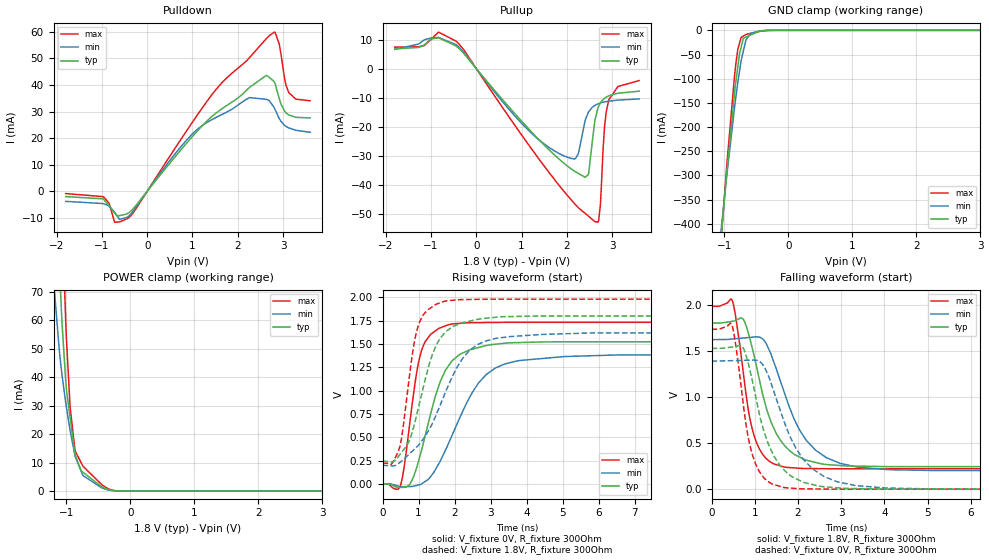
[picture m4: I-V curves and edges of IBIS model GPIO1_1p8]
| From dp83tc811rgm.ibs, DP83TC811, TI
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|   GPIO1_1p8 Model
[Model]   GPIO1_1p8
Model_type   I/O
Polarity   Non-Inverting
Enable   Active-Low
Vinl = 0.63
Vinh = 1.17
Vmeas = 0.9
Vref = 0
Cref = 2pF
Rref = 100000
|   typ   min   max
C_comp   7.7920pF   5.5675pF   10.3673pF
[Model spec]
|subparameter
Vinl   0.63   0.567   0.693
Vinh   1.17   1.053   1.287
| Where Nom  PVT is Nominal Process, 1.8V, 27C
|   Fast PVT is Strong Process,  1.98V, -40C
|   Slow PVT is Weak Process,   1.62V, 125C
[Voltage Range]   1.8   1.62   1.98
|Junction Temperature
[Temperature Range]   27   125   -40
[Pullup Reference]   1.8   1.62   1.98
[Pulldown Reference]   0   0   0
[Power Clamp Reference]   1.8   1.62   1.98
[GND Clamp Reference]   0   0   0
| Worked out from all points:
|   slope of the pulldown table from 0 to 0.27 V, typ, clamps not added: 46.9 ohm
|   slope of the pullup table from 0 to 0.27 V, typ, clamps not added: 53.6 ohm
|   GND clamp passes 1 mA (typ) near -0.41 V on its own axis
|   POWER clamp passes 1 mA (typ) near -0.41 V on its own axis
|   falling waveform, V_fixture 1.8V, R_fixture 300Ohm: 20-80 % time 599ps typ, 811ps min, 356ps max; typ from 1.8 V to 0.243 V
|   rising waveform, V_fixture 0V, R_fixture 300Ohm: 20-80 % time 706ps typ, 1.09ns min, 393ps max; typ from 0 V to 1.52 V
|   rising waveform, V_fixture 1.8V, R_fixture 300Ohm: 20-80 % time 673ps typ, 1.07ns min, 384ps max; typ from 0.243 V to 1.8 V
|   falling waveform, V_fixture 0V, R_fixture 300Ohm: 20-80 % time 592ps typ, 811ps min, 353ps max; typ from 1.52 V to 0 V
[Pulldown]
|   Voltage   I(typ)   I(min)   I(max)
-1.8V     -2.003mA   -3.807mA   -871.8uA
-952.2mV  -3.215mA   -4.752mA   -2.279mA
-720mV    -8.21mA    -7.846mA   -11.65mA
-390.6mV  -7.919mA   -9.075mA   -9.66mA
1.165V    23.73mA    24.11mA    30.11mA
2.261V    39.13mA    35.27mA    50.31mA
2.633V    43.65mA    34.6mA     57.5mA
2.806V    41.24mA    31.48mA    59.92mA
2.914V    35.03mA    27.45mA    55.52mA
3.038V    30.09mA    24.77mA    42.01mA
3.125V    28.76mA    23.85mA    37.24mA
3.6V      27.61mA    22.2mA     34.08mA
[GND Clamp]
|   Voltage   I(typ)   I(min)   I(max)
-1.8V     -1.617A    -1.421A    -1.801A
-1.13V    -546.6mA   -513.3mA   -570.5mA
-968.4mV  -303.6mA   -307.9mA   -289.4mA
-844.2mV  -135.1mA   -163.2mA   -98.54mA
-790.2mV  -75.61mA   -107.9mA   -39.81mA
-763.2mV  -48.67mA   -84.29mA   -26.44mA
-741.6mV  -36.91mA   -65.42mA   -15.75mA
-703.8mV  -16.33mA   -42.95mA   -11.89mA
-666mV    -14.15mA   -21.56mA   -8.729mA
-590.4mV  -9.772mA   -6.228mA   -6.206mA
-347.4mV  -341.4uA   -282.5uA   -494.2uA
3.6V      0A         0A         0A
[Pullup]
|   Voltage   I(typ)   I(min)   I(max)
-1.8V     6.759mA    6.611mA    7.381mA
-833.4mV  10.6mA     10.7mA     12.56mA
-444.6mV  7.764mA    8.247mA    9.418mA
1.732V    -29.81mA   -28.41mA   -38.29mA
2.191V    -35.53mA   -31.05mA   -46.86mA
2.407V    -37.45mA   -17.78mA   -49.9mA
2.482V    -36.21mA   -14.93mA   -50.89mA
2.687V    -13.63mA   -12.18mA   -52.94mA
2.741V    -11.86mA   -11.87mA   -47.25mA
2.839V    -10.19mA   -11.49mA   -19.37mA
2.925V    -9.409mA   -11.25mA   -11mA
3.6V      -7.807mA   -10.48mA   -4.149mA
[POWER Clamp]
|   Voltage   I(typ)   I(min)   I(max)
-1.8V     670.8mA    497.2mA    807.9mA
-1.184V   129.3mA    70.13mA    198.4mA
-1.087V   68.67mA    44.65mA    114.6mA
-1.066V   58.56mA    40.52mA    97.74mA
-1.012V   39.41mA    31.41mA    60.89mA
-995.4mV  35.1mA     28.97mA    52.43mA
-941.4mV  25.86mA    21.28mA    29.56mA
-860.4mV  12.59mA    12.01mA    13.99mA
-741.6mV  6.6mA      5.425mA    8.724mA
-444.6mV  1.42mA     1.065mA    2.177mA
-180mV    12.02uA    16.35uA    15.6uA
3.6V      0A         0A         0A
[Ramp]
R_load = 300
|   typ   min   max
dV/dt_r   0.914819/7.04525e-10   0.831976/1.07942e-09   1.03915/3.921e-10
dV/dt_f   0.934/5.95666e-10   0.852196/8.00312e-10   1.05541/3.5521e-10
[Falling Waveform]
V_fixture = 1.8V
V_fixture_min = 1.62V
V_fixture_max = 1.98V
R_fixture = 300Ohm
C_fixture = 0F
|   Time   V(typ)   V(min)   V(max)
0s        1.8V       1.62V      1.98V
478.9ps   1.819V     1.627V     2.044V
742.1ps   1.835V     1.638V     1.233V
872ps     1.657V     1.644V     800.6mV
1.044ns   1.321V     1.651V     501.1mV
1.284ns   849.9mV    1.557V     323.6mV
1.652ns   494.3mV    1.09V      242.8mV
2.406ns   289.3mV    422.4mV    223mV
3.4ns     249.4mV    237.7mV    221.1mV
20ns      243.3mV    199.6mV    220.9mV
[Rising Waveform]
V_fixture = 0V
V_fixture_min = 0V
V_fixture_max = 0V
R_fixture = 300Ohm
C_fixture = 0F
|   Time   V(typ)   V(min)   V(max)
0s        27.15uV    65.29uV    36.54uV
489.2ps   -37.9mV    -30.23mV   -27.51mV
811.2ps   33.75mV    -27.71mV   823.1mV
988.9ps   230.6mV    -12.52mV   1.283V
1.128ns   430.5mV    11.88mV    1.477V
1.468ns   942.4mV    153.5mV    1.64V
1.84ns    1.271V     442.3mV    1.707V
2.67ns    1.461V     1.084V     1.727V
3.809ns   1.514V     1.322V     1.731V
20ns      1.525V     1.387V     1.732V
[Rising Waveform]
V_fixture = 1.8V
V_fixture_min = 1.62V
V_fixture_max = 1.98V
R_fixture = 300Ohm
C_fixture = 0F
|   Time   V(typ)   V(min)   V(max)
0s        243.3mV    199.6mV    220.9mV
244.6ps   236.1mV    193.7mV    212.5mV
474.2ps   310.8mV    227.9mV    389.6mV
845.3ps   584.6mV    357.7mV    1.433V
1.021ns   858.1mV    426.5mV    1.729V
1.379ns   1.382V     645.1mV    1.897V
1.696ns   1.604V     935.5mV    1.954V
2.406ns   1.742V     1.426V     1.975V
3.57ns    1.793V     1.579V     1.979V
20ns      1.8V       1.62V      1.98V
[Falling Waveform]
|Gnd
V_fixture = 0V
V_fixture_min = 0V
V_fixture_max = 0V
R_fixture = 300Ohm
C_fixture = 0F
|   Time   V(typ)   V(min)   V(max)
0s        1.525V     1.387V     1.732V
463.7ps   1.539V     1.392V     1.79V
714ps     1.545V     1.395V     997.3mV
839.4ps   1.379V     1.397V     582mV
1.015ns   1.015V     1.399V     278.4mV
1.314ns   487.9mV    1.23V      80.69mV
1.652ns   220mV      767.5mV    20.15mV
2.339ns   49.66mV    219mV      2.315mV
3.34ns    6.494mV    38.71mV    240.3uV
20ns      27.15uV    65.28uV    36.09uV
